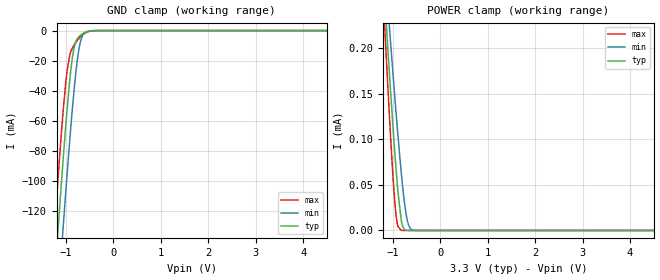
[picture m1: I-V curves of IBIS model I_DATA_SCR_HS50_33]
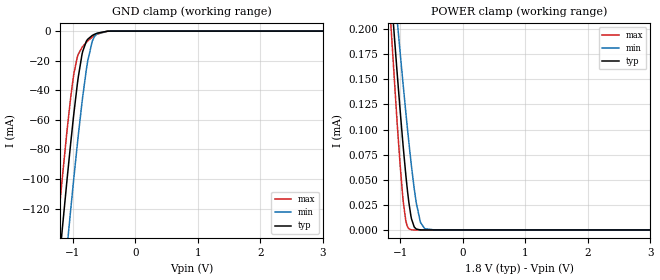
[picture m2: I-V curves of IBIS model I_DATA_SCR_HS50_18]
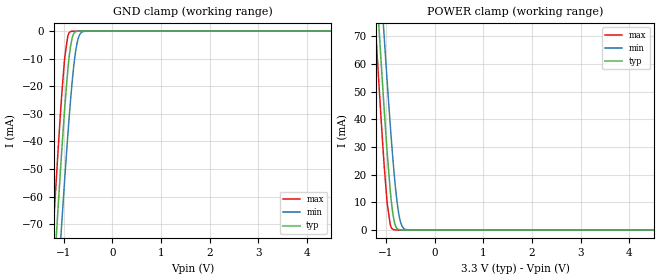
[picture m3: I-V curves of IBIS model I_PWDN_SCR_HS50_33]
| Texas Instruments Incorporated
| DS90UR906Q
| 5-65MHz 24-bit Color Link II Serializer and Deserializer
| Marketing part#   Voltage Range   Package-type   Temperature
| DS90UR916QSQE   1.71V - 3.6V   60-Pin LLP   -40 to 105C
| DS90UR916QSQ   1.71V - 3.6V   60-Pin LLP   -40 to 105C
| DS90UR916QSQX   1.71V - 3.6V   60-Pin LLP   -40 to 105C
[IBIS Ver]   4.0
[File name]   ds90ur916.ibs
[File Rev]   1.0
[Date]   03/27/2012
[Source]   Model built from TISPICE simulations at:
   Texas Instruments Incorporated.
   WEBENCH DESIGN CENTER
   12500 TI Blvd
   Dallas, TX -75243
   For Support e-mail: elab_scm_ibis@list.ti.com
[Notes]   Rev 1.0: 03/27/2012
   - Initial version of the IBIS model
   - All models are generated in Spectre
   - ccomp is listed in numerical order, for PVT information,
   please check notes above ccomp keyword for each model
   - All non-monotonic warnings can be ignored as per buffer behavior
[Disclaimer] This product is designed as an aid for customers of Texas Instruments.
   No warranties, either expressed or implied, with respect to this third
   party software (if any) or with respect to its fitness for any
   particular purpose is claimed by Texas Instruments or the author. The
   software (if any) is provided solely on an "as is" basis. The entire
   risk as to its quality and performance is with the customer
[Copyright]   (C)Copyright 2012 Texas Instruments Incorporated.
   All rights reserved.
[Component]   DS90UR916Q
[Manufacturer]  Texas Instruments, Inc.
[Package]   |60-pin LLP 9.0X9.0X0.8mm
|   typ   min   max
R_pkg   0   0   0
L_pkg   0   0   0
C_pkg   0   0   0
[Pin]   signal_name   model_name   R_pin   L_pin   C_pin
1   NC   NC
2   SDA   IO_SMBUS_LVCMOS_HS50
3   SCL   IO_SMBUS_LVCMOS_HS50
4   VDDSC   POWER
5   CLKOUT   IO_CLK_50_HS50
6   CO1   IO_DATA_50_HS50
7   CO3   IO_DATA_50_HS50
8   CO2   IO_DATA_50_HS50
9   DO23_CONFIG[0]  IO_DATA_50_HS50
10   DO22_CONFIG[1]  IO_DATA_50_HS50
11   DO21_OSCLKOUT   IO_DATA_50_HS50
12   DO20_LFMODE   IO_DATA_50_HS50
13   VDDIO   POWER
14   DO19_OSDATA   IO_DATA_50_HS50
15   NC   NC
16   NC   NC
17   DO18_OSSSEL   IO_DATA_50_HS50
18   DO17_RFB   IO_DATA_50_HS50
19   DO16   IO_DATA_50_HS50
20   DO15_EQ3   IO_DATA_50_HS50
21   DO14_EQ2   IO_DATA_50_HS50
22   DO13_EQ1   IO_DATA_50_HS50
23   DO12_EQ0   IO_DATA_50_HS50
24   VDDIO   POWER
25   DO11   IO_DATA_50_HS50
26   DO10_OSCSEL2   IO_DATA_50_HS50
27   DO9_OSCSEL1   IO_DATA_50_HS50
28   DO8_OSCSEL0   IO_DATA_50_HS50
29   VDDL   POWER
30   NC   NC
31   NC   NC
32   LOCK   IO_DATA_50_HS50
33   DO7   IO_DATA_50_HS50
34   DO6_SSC3   IO_DATA_50_HS50
35   DO5_SSC2   IO_DATA_50_HS50
36   DO4_SSC1   IO_DATA_50_HS50
37   DO3_SSC0   IO_DATA_50_HS50
38   VDDIO   POWER
39   DO2   IO_DATA_50_HS50
40   DO1   IO_DATA_50_HS50
41   DO0   IO_DATA_50_HS50
42   PASS_OPLOW   IO_DATA_50_HS50
43   VDDR   POWER
44   BISTEN   I_DATA_SCR_HS50
45   NC   NC
46   NC   NC
47   RES   NC
48   VDDIR   POWER
49   RIN+   NC
50   RIN-   NC
51   CMF   NC
52   ROUT+   NC
53   ROUT-   NC
54   VDDCMLO   POWER
55   VDDR   POWER
56   ID[x]   NC
57   VDDPR   POWER
58   VDDSC   POWER
59   PDB   I_PWDN_SCR_HS50
60   NC   NC
61   DAP   GND
[Package Model] llp60_DS90UR906QSQ
[Diff pin]  inv_pin  vdiff  tdelay_typ  tdelay_min  tdelay_max
49   50   1.0   0.0s   0.0s   0.0s
52   53   0.0   0.0s   0.0s   0.0s
[Model Selector]   I_DATA_SCR_HS50
I_DATA_SCR_HS50_33   I_DATA_SCR_HS50 input with VDD=3.3V
I_DATA_SCR_HS50_18   I_DATA_SCR_HS50 input with VDD=1.8V
[Model Selector]   I_PWDN_SCR_HS50
I_PWDN_SCR_HS50_33   I_PWDN_SCR_HS50 input with VDD=3.3V
I_PWDN_SCR_HS50_18   I_PWDN_SCR_HS50 input with VDD=1.8V
[Model Selector]   IO_DATA_50_HS50
IO_DATA_50_HS50_33   IO_DATA_50_HS50 with VDD=3.3V
IO_DATA_50_HS50_18   IO_DATA_50_HS50 with VDD=1.8V
[Model Selector]   IO_CLK_50_HS50
IO_CLK_50_HS50_33   IO_CLK_50_HS50 with VDD=3.3V
IO_CLK_50_HS50_18   IO_CLK_50_HS50 with VDD=1.8V
[Model Selector]   IO_SMBUS_LVCMOS_HS50
IO_SMBUS_LVCMOS_HS50_33_HI   IO_SMBUS_HS50 HI DRIVE with VDD=3.3V
IO_SMBUS_LVCMOS_HS50_33_LO   IO_SMBUS_HS50 LO DRIVE with VDD=3.3V
IO_SMBUS_LVCMOS_HS50_18_HI   IO_SMBUS_HS50 HI DRIVE with VDD=1.8V
IO_SMBUS_LVCMOS_HS50_18_LO   IO_SMBUS_HS50 LO DRIVE with VDD=1.8V
[Define Package Model]  llp60_DS90UR906QSQ
[Manufacturer]  Texas Instruments, Inc.
[OEM]  Texas Instruments, Inc.
[Description]  None
[Number Of Pins]  49
[Pin Numbers]
61   | 61 = DAP
2   | 2 = L2
3   | 3 = L3
4   | 4 = L4
5   | 5 = L5
6   | 6 = L6
7   | 7 = L7
8   | 8 = L8
9   | 9 = L9
10   | 10 = L10
11   | 11 = L11
12   | 12 = L12
13   | 13 = L13
14   | 14 = L14
18   | 18 = L18
19   | 19 = L19
20   | 20 = L20
21   | 21 = L21
22   | 22 = L22
23   | 23 = L23
24   | 24 = L24
25   | 25 = L25
26   | 26 = L26
27   | 27 = L27
28   | 28 = L28
29   | 29 = L29
34   | 34 = L34
35   | 35 = L35
36   | 36 = L36
37   | 37 = L37
38   | 38 = L38
39   | 39 = L39
40   | 40 = L40
41   | 41 = L41
42   | 42 = L42
43   | 43 = L43
44   | 44 = L44
48   | 48 = L48
49   | 49 = L49
50   | 50 = L50
51   | 51 = L51
52   | 52 = L52
53   | 53 = L53
54   | 54 = L54
55   | 55 = L55
56   | 56 = L56
57   | 57 = L57
58   | 58 = L58
59   | 59 = L59
[Model Data]
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[End Model Data]
[End Package Model]
| Models and submodels in the file (12): I_DATA_SCR_HS50_33 (Input), I_DATA_SCR_HS50_18 (Input), I_PWDN_SCR_HS50_33 (Input), I_PWDN_SCR_HS50_18 (Input), IO_DATA_50_HS50_33 (I/O), IO_DATA_50_HS50_18 (I/O), IO_CLK_50_HS50_33 (I/O), IO_CLK_50_HS50_18 (I/O), IO_SMBUS_LVCMOS_HS50_33_HI (I/O), IO_SMBUS_LVCMOS_HS50_33_LO (I/O), IO_SMBUS_LVCMOS_HS50_18_HI (I/O), IO_SMBUS_LVCMOS_HS50_18_LO (I/O)
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|   Model I_DATA_SCR_HS50_33
[Model] I_DATA_SCR_HS50_33
Model_type Input
Vinl =   0.8
Vinh =   2.0
|   typ   min   max
|   (nom)   (slow)   (fast)
C_comp   0.3665pF   0.3665pF   0.3665pF
[Temperature Range]   25.000   105.000   -40.000
[Voltage Range]   3.300V   3.0000V   3.6000V
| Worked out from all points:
|   GND clamp passes 1 mA (typ) near -0.58 V on its own axis
|   POWER clamp passes 1 mA (typ) near -2.02 V on its own axis
[GND Clamp]
|   Voltage   I(typ)   I(min)   I(max)
-3.3V     -1.166A    -1.209A    -1.134A
-1.32V    -202.1mA   -249mA     -167.1mA
-1.241V   -165.6mA   -212.4mA   -130.7mA
-1.142V   -121mA     -167.4mA   -86.89mA
-1.063V   -86.78mA   -132.3mA   -54.56mA
-983.4mV  -54.93mA   -98.36mA   -28.27mA
-924mV    -33.98mA   -74.16mA   -16.74mA
-825mV    -10.8mA    -38mA      -9.446mA
-755.7mV  -5.134mA   -18.34mA   -6.356mA
-696.3mV  -3.098mA   -7.601mA   -4.22mA
-567.6mV  -815.5uA   -746uA     -1.217mA
6.59V     0A         0A         0A
[POWER Clamp]
|   Voltage   I(typ)   I(min)   I(max)
-3.3V     2.159mA    1.892mA    2.559mA
-1.191V   270.3uA    306.6uA    243.1uA
-1.132V   220.6uA    264.4uA    182.9uA
-1.063V   164.1uA    216.1uA    115.7uA
-993.3mV  110.2uA    168.9uA    55.28uA
-933.9mV  67.72uA    129.8uA    16.89uA
-894.3mV  42.8uA     104.8uA    4.336uA
-825mV    11.61uA    64.2uA     166.8nA
-755.7mV  1.271uA    30.48uA    2.122nA
-696.3mV  130.3nA    11.15uA    0A
-557.7mV  0A         260.4nA    0A
6.59V     0A         0A         0A
|   Model I_DATA_SCR_HS50_18
[Model] I_DATA_SCR_HS50_18
Model_type Input
Vinl =   0.63
Vinh =   1.17
|   typ   min   max
|   (nom)   (fast)   (slow)
C_comp   0.5298pF   0.3665pF   0.5298pF
[Temperature Range]   25.000   105.000   -40.000
[Voltage Range]   1.800V   1.7100V   1.8900V
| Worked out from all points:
|   GND clamp passes 1 mA (typ) near -0.56 V on its own axis
[GND Clamp]
|   Voltage   I(typ)   I(min)   I(max)
-1.8V     -430.9mA   -477mA     -396.6mA
-1.238V   -164.5mA   -211.3mA   -129.6mA
-1.174V   -135.2mA   -181.7mA   -100.7mA
-1.093V   -99.54mA   -145.4mA   -66.37mA
-1.039V   -76.81mA   -121.8mA   -45.69mA
-984.6mV  -55.39mA   -98.86mA   -28.59mA
-930.6mV  -36.12mA   -76.78mA   -17.61mA
-855mV    -15.77mA   -48.21mA   -11.06mA
-763.2mV  -5.498mA   -20.14mA   -6.658mA
-687.6mV  -2.877mA   -6.556mA   -3.945mA
-450mV    -97.64uA   -77.9uA    -176.8uA
3.595V    0A         0A         0A
[POWER Clamp]
|   Voltage   I(typ)   I(min)   I(max)
-1.8V     803.7uA    754.7uA    897.4uA
-1.157V   241.8uA    282.5uA    208.5uA
-1.055V   157.9uA    210.7uA    108.4uA
-1.012V   124.1uA    181.2uA    70.17uA
-952.2mV  80.3uA     141.7uA    26.6uA
-914.4mV  55uA       117.4uA    9.25uA
-865.8mV  27.6uA     87.52uA    1.228uA
-822.6mV  10.92uA    62.89uA    149.1nA
-747mV    921.8nA    26.99uA    1.513nA
-682.2mV  75.41nA    8.215uA    0A
-612mV    3.441nA    1.296uA    0A
3.595V    0A         0A         0A
|   Model I_PWDN_SCR_HS50_33
[Model] I_PWDN_SCR_HS50_33
Model_type Input
Vinl =   0.8
Vinh =   2.0
|   typ   min   max
|   (nom)   (fast)   (slow)
C_comp   0.3665pF   0.3665pF   0.5298pF
[Temperature Range]   25.000   105.000   -40.000
[Voltage Range]   3.300V   3.0000V   3.6000V
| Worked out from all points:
|   GND clamp passes 1 mA (typ) near -0.79 V on its own axis
|   POWER clamp passes 1 mA (typ) near -0.79 V on its own axis
[GND Clamp]
|   Voltage   I(typ)   I(min)   I(max)
-3.3V     -740.6mA   -745.8mA   -738.2mA
-1.211V   -92.27mA   -118mA     -71.83mA
-1.191V   -86.5mA    -112.3mA   -65.95mA
-1.112V   -63.85mA   -90.11mA   -43.04mA
-1.043V   -44.84mA   -71.14mA   -24.45mA
-973.5mV  -27.25mA   -52.87mA   -9.257mA
-914.1mV  -14.38mA   -38.09mA   -1.938mA
-854.7mV  -5.279mA   -24.66mA   -158.3uA
-785.4mV  -769.6uA   -11.9mA    -11.81uA
-726mV    -91.41uA   -4.691mA   -6.467uA
-577.5mV  -3.449uA   -99.25uA   -4.919uA
6.59V     0A         0A         0A
[POWER Clamp]
|   Voltage   I(typ)   I(min)   I(max)
-3.3V     739mA      744.2mA    736.5mA
-1.211V   92.02mA    117.6mA    71.62mA
-1.191V   86.27mA    112mA      65.75mA
-1.112V   63.66mA    89.86mA    42.89mA
-1.043V   44.7mA     70.93mA    24.36mA
-973.5mV  27.14mA    52.7mA     9.21mA
-914.1mV  14.31mA    37.95mA    1.931mA
-854.7mV  5.248mA    24.55mA    164.4uA
-785.4mV  767.3uA    11.83mA    19.72uA
-726mV    94.5uA     4.66mA     14.93uA
-577.5mV  8.162uA    100.4uA    14.65uA
6.59V     0A         0A         0A
